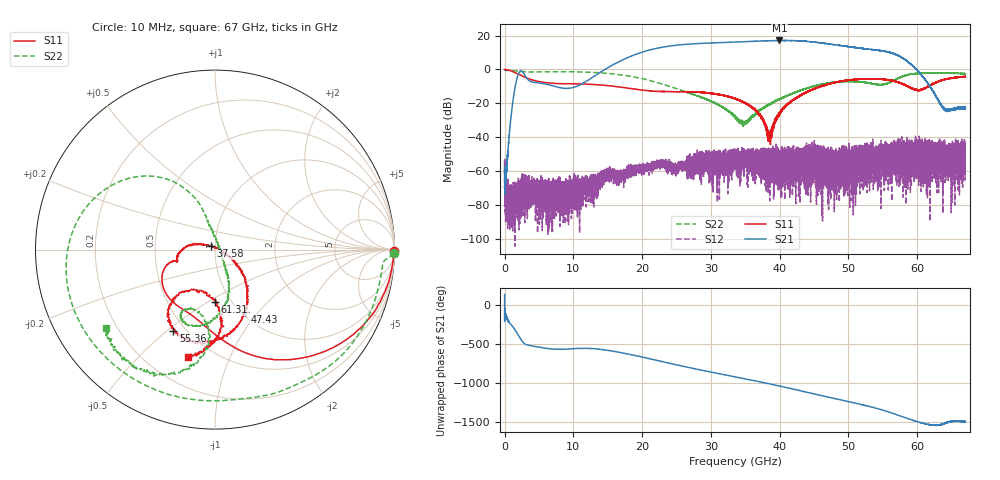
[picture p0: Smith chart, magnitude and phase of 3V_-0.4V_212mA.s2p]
! MARKI MICROWAVE INC.
! Date:  10/21/2020
! Model Number:  AMM-7210CH
! Description:  2-port Small Signal S-parameter data for AMM-7210CH
! Frequency Range:  10 MHz to 67 GHz
! Port Configuration:  PORT 1: Input
!  PORT 2: Output
! Bias Condition: Vd = +3.0V, Vg = -0.4V
! AMM-7210CH s2p files are only valid for small signal conditions (below -10 dBm input power)
# Hz S  dB  R 50
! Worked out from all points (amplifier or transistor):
!   20001 points, 10 MHz to 67 GHz, reference 50 ohm
!   highest |S21| = 17.1 dB at 39.96 GHz (marker M1)
!   |S21| within 3 dB of that: 24.59 GHz to 48.81 GHz (24.22 GHz wide, 66 % of centre)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
!   unconditionally stable (mu >= 1): start of sweep to end of sweep
!   at 11.17 GHz: K = 947.32, MAG = -2.7 dB, |S12| = -68.9 dB
!   at 33.51 GHz: K = 37.01, MAG = 16.3 dB, |S12| = -53.8 dB
!   at 67 GHz: K = 406.04, MAG = -16.9 dB, |S12| = -46.9 dB
!   S11 on the Smith chart (normalised r, x): 10 MHz: open; 37.58 GHz: 0.95, +0.04; 47.43 GHz: 1.05, -0.86; 55.36 GHz: 0.43, -0.52; 61.31 GHz: 0.84, -0.54; 67 GHz: 0.38, -0.70
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1e7  -0.03 -0.4  -57.39 130.0  -53.88 -148.7  -0.02 -1.2
2.22402e9  -3.22 -62.5  -1.21 -61.5  -73.34 -143.5  -1.17 -61.6
1.117723e10  -8.58 -132.5  -8.70 162.8  -64.47 -167.4  -1.48 -168.6
1.705226e10  -10.56 -160.2  5.42 105.9  -62.54 129.3  -3.28 149.4
1.991608e10  -12.14 -164.5  10.09 53.1  -58.74 133.6  -5.35 130.7
2.234112e10  -13.01 -162.8  12.68 4.9  -55.85 89.9  -7.96 118.0
2.472261e10  -13.20 -163.3  14.21 -42.5  -56.71 92.4  -10.99 109.5
2.776731e10  -13.34 -167.9  15.23 -100.2  -55.27 66.3  -15.24 105.2
3.092588e10  -14.76 -178.9  15.77 -156.5  -54.15 84.6  -20.59 97.3
3.3505e10  -17.20 169.4  16.19 158.7  -53.76 24.2  -27.96 73.0
3.758134e10  -30.28 141.3  16.83 86.4  -52.75 -48.0  -22.81 -52.9
3.995614e10  -25.99 -14.4  17.14 41.9  -51.42 -92.7  -17.51 -62.5
4.226394e10  -16.96 -35.3  16.99 -3.8  -54.53 -164.5  -13.51 -68.4
4.467223e10  -12.00 -46.9  16.38 -52.9  -46.65 -140.8  -10.26 -79.5
4.743222e10  -8.28 -64.0  14.93 -107.6  -59.00 -156.6  -7.86 -94.1
5.109322e10  -5.92 -90.3  12.92 -179.5  -54.62 -19.3  -7.18 -113.9
5.351491e10  -5.63 -105.2  11.66 129.6  -57.62 -36.7  -8.50 -116.6
5.536049e10  -5.89 -117.3  10.67 83.5  -43.05 -157.3  -8.63 -102.1
5.583612e10  -6.20 -120.3  10.23 70.1  -47.27 165.1  -7.89 -98.0
5.869659e10  -10.41 -128.8  4.25 -17.1  -46.02 38.2  -3.08 -104.5
6.130585e10  -10.67 -89.8  -6.83 -84.4  -52.17 -158.8  -2.05 -121.9
6.7e10  -4.37 -105.0  -22.45 -53.0  -46.89 -94.6  -2.49 -144.6
